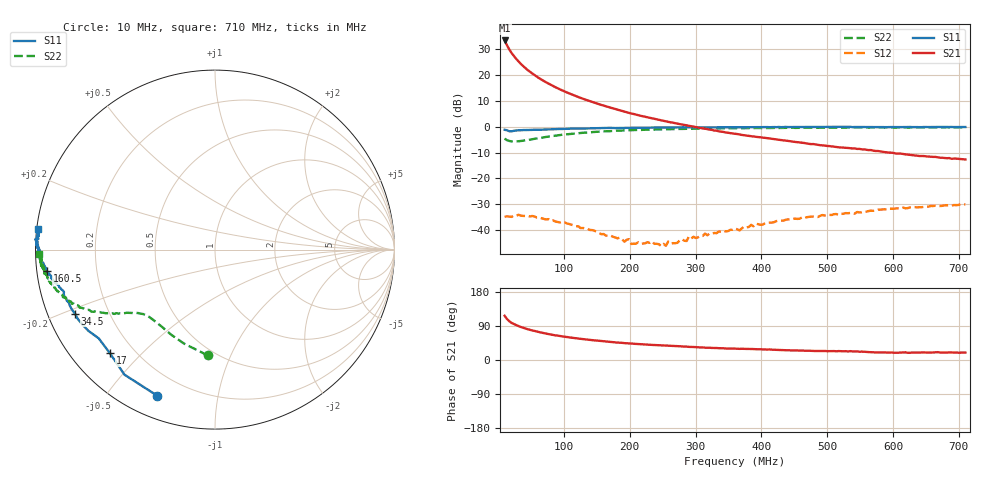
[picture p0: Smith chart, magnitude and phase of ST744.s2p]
!  POLYFET RF DEVICES
!  S PARAMETERS FOR
!  ST744
!  VDS=50, IDQ=400MA
# MHZ S MA R 50
! Freq=Mhz Mag[s11] Ang[s11] Mag[s21] Ang[s21] Mag[s12] Ang[s12] Mag[s22] Ang[s22]
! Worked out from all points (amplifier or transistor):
!   201 points, 10 MHz to 710 MHz, reference 50 ohm
!   highest |S21| = 33.5 dB at 10 MHz (marker M1)
!   |S21| within 3 dB of that: start of sweep to 16.05 MHz
!   unconditionally stable (mu >= 1): nowhere
!   at 125.5 MHz: K = 0.10, MSG = 25.2 dB, |S12| = -39.3 dB
!   at 360 MHz: K = 0.42, MSG = 18.4 dB, |S12| = -39.4 dB
!   at 710 MHz: K = 0.67, MSG = 8.7 dB, |S12| = -30.1 dB
!   S11 on the Smith chart (normalised r, x): 10 MHz: 0.10, -0.67; 17 MHz: 0.11, -0.41; 34.5 MHz: 0.08, -0.22; 160.5 MHz: 0.03, -0.06; 710 MHz: 0.00, +0.06
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10  0.875 -111.6  47.2 116.7  0.01806 29.6  0.5907 -94.0
13.5  0.8603 -125.9  38.36 108.4  0.01839 21.1  0.5514 -108.2
17  0.8222 -135.5  31.74 102.4  0.01824 15.9  0.5329 -117.5
20.5  0.815 -142.7  27.05 98.0  0.01793 11.2  0.5225 -124.0
24  0.8381 -147.3  23.74 95.0  0.01903 9.3  0.5202 -128.5
27.5  0.8487 -150.5  20.88 92.2  0.01886 4.2  0.5218 -131.9
31  0.857 -153.4  18.58 89.7  0.01974 3.4  0.525 -134.5
34.5  0.8577 -155.4  16.64 87.1  0.01901 -1.6  0.5309 -136.6
41.5  0.8668 -158.9  13.78 83.1  0.01873 -2.9  0.5479 -139.4
48.5  0.8734 -161.0  11.68 79.6  0.01827 -5.8  0.5653 -141.4
59  0.878 -163.7  9.397 75.1  0.01743 -10.9  0.5953 -143.6
69.5  0.8852 -165.6  7.717 71.0  0.01649 -14.0  0.6261 -145.3
80  0.8927 -167.0  6.516 67.3  0.01509 -16.0  0.6544 -147.2
94  0.9088 -168.1  5.322 63.3  0.01398 -20.3  0.6911 -149.2
129  0.9251 -170.9  3.49 55.2  0.01095 -21.2  0.7662 -153.1
160.5  0.9446 -172.7  2.587 49.4  0.00835 -13.4  0.8178 -156.7
199  0.956 -174.6  1.856 43.7  0.00663 2.6  0.8596 -160.1
244.5  0.9694 -176.4  1.364 38.8  0.0053 30.9  0.8884 -163.6
360  0.9827 -179.5  0.7343 29.9  0.0107 82.0  0.9421 -169.5
479  0.9961 177.8  0.4632 23.9  0.01816 94.8  0.9609 -173.4
594.5  0.9903 175.3  0.3161 19.6  0.02594 98.0  0.9695 -176.7
710  0.9908 173.3  0.2329 19.5  0.03134 104.0  0.9781 -178.7
